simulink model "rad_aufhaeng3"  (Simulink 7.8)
settings: Solver=ode45  StartTime=0.0  StopTime=10.0  RelTol=1e-3
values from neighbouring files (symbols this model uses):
  a1 = subplot(311), plot(t, vy-vb)    [coulomb_10.m]    (also in coulomb_11.m; coulomb_2.m = subplot(311),  plot(t, y1); coulomb_3.m = subplot(311),  plot(t, y1); coulomb_5.m = subplot(311),  plot(t, y1))
  a2 = subplot(312), plot(t, y)    [coulomb_10.m]    (also in coulomb_11.m; coulomb_2.m = subplot(312),  plot(t, y2); coulomb_3.m = subplot(312),  plot(t, y2); coulomb_5.m = subplot(312),  plot(t, y2))
  b1 = b{1}    [rad_aufhaeng_3.m]    (also in rad_aufhaeng_4.m; unwucht_2.m = b1{:})
  b2 = b{2}    [rad_aufhaeng_3.m]    (also in rad_aufhaeng_4.m)
  C = [c -c;-c ct+c]    [rad_aufhaeng_1.m]    (also in rad_aufhaeng_2.m; rad_aufhaeng_3.m; rad_aufhaeng_4.m; suspension_1.m = [c*(a^2 + (L-a)^2) c*L -c*a c*(L-a))
  K = [k -k; -k kt+k]    [rad_aufhaeng_1.m]    (also in rad_aufhaeng_2.m; rad_aufhaeng_3.m; rad_aufhaeng_4.m; suspension_1.m = [k*(a^2+(L-a)^2) k*L -k*a k*(L-a))
  M = [ms 0;0 ma]    [rad_aufhaeng_1.m]    (also in rad_aufhaeng_2.m; rad_aufhaeng_3.m; rad_aufhaeng_4.m; suspension_1.m = [I 0 0 0;0 ms 0 0;0 0 ma 0;0 0 0 ma])
  xv0 = [X(:,1),X(:,2),X(:,3),X(:,4);     X(:,1)*e(1),X(:,2)*e(2),X(:,3)*e(3),X(:,4)*e(4)]*p'    [rad_aufhaeng_2.m]    (also in rad_aufhaeng_3.m = [0.2; 0; 0; 0])

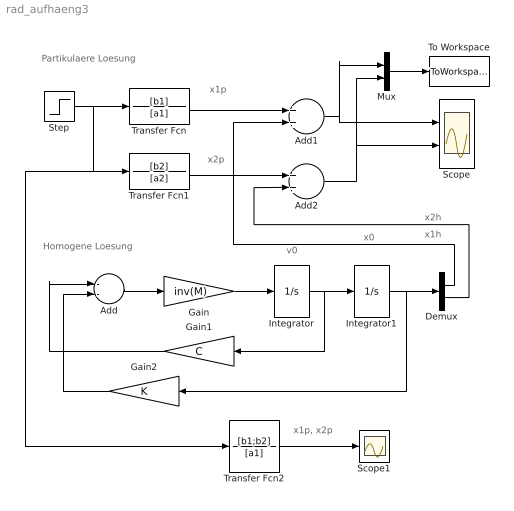
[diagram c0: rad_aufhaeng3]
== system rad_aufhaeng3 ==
  note: x1p, x2p
  note: x0
  note: v0
  note: x1h
  note: x2h
  note: Homogene Loesung
  note: Partikulaere Loesung
  note: x2p
  note: x1p
  Add : Sum  Inputs=--
  Add1 : Sum
  Add2 : Sum
  Demux : Demux  Outputs=2
  Gain : Gain  Gain=inv(M)  Multiplication=Matrix(K*u)
  Gain1 : Gain  Gain=C  Multiplication=Matrix(K*u)
  Gain2 : Gain  Gain=K  Multiplication=Matrix(K*u)
  Integrator : Integrator  InitialCondition=xv0(3:4,1)
  Integrator1 : Integrator  InitialCondition=xv0(1:2,1)
  Mux : Mux  Inputs=2
  Scope : Scope  NumInputPorts=2
  Scope1 : Scope
  Step : Step  Time=0  SampleTime=0
  To Workspace : ToWorkspace  VariableName=x  SampleTime=-1  SaveFormat=Structure With Time
  Transfer Fcn : TransferFcn  Numerator=[b1]  Denominator=[a1]
  Transfer Fcn1 : TransferFcn  Numerator=[b2]  Denominator=[a2]
  Transfer Fcn2 : TransferFcn  Numerator=[b1;b2]  Denominator=[a1]
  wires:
  Add/1 -> Gain/1
  Gain/1 -> Integrator/1
  Integrator/1 -> Gain1/1, Integrator1/1
  Gain1/1 -> Add/1
  Gain2/1 -> Add/2
  Integrator1/1 -> Demux/1, Gain2/1
  Transfer Fcn1/1 -> Add2/1
  Demux/2 -> Add2/2
  Transfer Fcn/1 -> Add1/1
  Demux/1 -> Add1/2
  Add2/1 -> Mux/2, Scope/2
  Add1/1 -> Mux/1, Scope/1
  Mux/1 -> To Workspace/1
  Transfer Fcn2/1 -> Scope1/1
  Step/1 -> Transfer Fcn2/1, Transfer Fcn1/1, Transfer Fcn/1
